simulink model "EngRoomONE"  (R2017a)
settings: Solver=VariableStepAuto  StartTime=0.0  StopTime=10.0  RelTol=1e-3
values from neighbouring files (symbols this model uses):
  EngDat = engine_pre()    [run_master.m]    (also in engine_pre.m = [MCR1, BSFC1, x)
undefined symbols (not defined in the file or in its folder): num

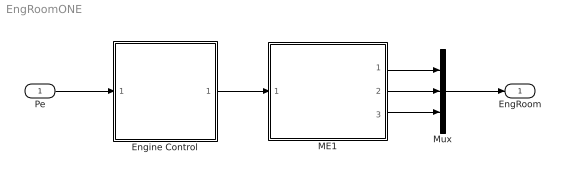
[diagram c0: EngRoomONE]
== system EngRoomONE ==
  Pe : Inport
  Engine Control : MATLAB Function  TreatAsAtomicUnit=on
  ME1 : MATLAB Function  TreatAsAtomicUnit=on
  Mux : Mux  Inputs=3
  EngRoom : Outport
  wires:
  Pe/1 -> Engine Control/1(Pe)
  Engine Control/1(P1) -> ME1/1("Pb ")
  ME1/1(fuel_cons) -> Mux/1
  ME1/2(Pb) -> Mux/2
  ME1/3(x) -> Mux/3
  Mux/1 -> EngRoom/1

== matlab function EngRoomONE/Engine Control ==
function P1   = fcn(Pe,EngDat)
%take in the total propulsive powering need
%find the optimal settings so that each engine runs close to optimum
%output the load (and rpm) for each engine

%Pe is the required effective power to overcome resistance, the break power
%needed from the engineroom depends on the efficiency of the propulsion
%system, which in turn depends on the configuration of the engines and
%propulsors

%capacity of each engine
PMCR1=EngDat(1,1);
%% Convert Pe into Pb required from the machinery
%eta_D = 0.55;
%eta_M = 0.95*0.98;
eta_T = 0.7;%eta_D* eta_M;   %Total efficiency
Pb = (Pe/eta_T); %kW
    
    
%If the ship only has one engine then this provides all the load
   P1=Pb;
   
end

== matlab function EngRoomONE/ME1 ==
function [fuel_cons, Pb, x] = fcn(Pb, num, EngDat)

%take in break power need [W], output fuel consumption [kg/h], Pb [W], and
%loading degree x [%]

PMCR=EngDat(1,1);

BSFC=EngDat(1,2); %g/kWh
delta_BSFC = 0;%6610.6*x^6 - 20524*x^5 + 23791*x^4 - 11985*x^3 + 1803.2*x^2 + 340.12*x - 36.733;


x = Pb/PMCR; %percentage of maximum
Pb=Pb*1; % [W] 
fuel_cons = ((delta_BSFC+BSFC)*(Pb/1000))/(1000); %[kg/hour]


end
